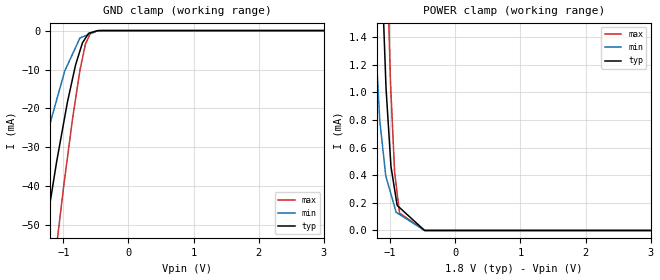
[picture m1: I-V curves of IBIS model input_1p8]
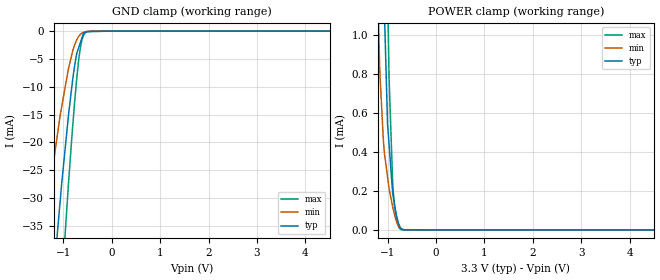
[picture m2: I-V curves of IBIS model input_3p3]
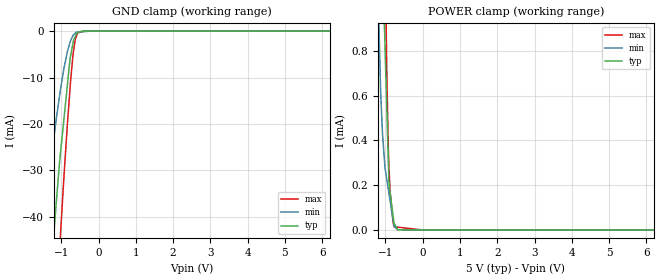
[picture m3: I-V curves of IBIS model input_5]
|Texas Instruments Incorporated
| Low-Power, 12-Bit, 1-MHz, Single/Dual Unipolar Input,
| ADCs with Serial Interface
| Marketing part#   Digital Voltage Range   Package-type   #pins
| ADS7229IPW   1.65V - 5.5V   TSSOP   16
| ADS7229IPWG4   1.65V - 5.5V   TSSOP   16
| ADS7229IPWR   1.65V - 5.5V   TSSOP   16
| ADS7229IPWRG4   1.65V - 5.5V   TSSOP   16
| ADS7229IRSAR   1.65V - 5.5V   QFN   16
| ADS7229IRSARG4   1.65V - 5.5V   QFN   16
| ADS7229IRSAT   1.65V - 5.5V   QFN   16
| ADS7229IRSATG4   1.65V - 5.5V   QFN   16
[IBIS Ver]   3.2
[File name]   ads7229.ibs
|SIMDE Ver   V3.0 - 201101 - RHL4 - Build 457
[File Rev]   1.0
[Date]   5/3/2011
[Source]
| Texas Instruments Incorporated.
| Analog-eLab Design Center, HPA
| 12500 TI Blvd
| Dallas, TX -75243
| e-mail: elab_ibis@list.ti.com
| -Model generated from simulations in TISPICE
[Notes]   Revision History:
| Rev 1.0: 5/3/2011
| - Initial version of the model
| - Model generated from simulations in TISPICE
| - Model matched to SPICE simulation
| - C_comp although listed in numerical order of value are
|   obtained from varying PVT conditions. For PVT conditions for
|   each specific value refer the buffer description under
|   respective [Model]. IBIS model user is responsible for using
|   appropriate C_comp to simulate for Signal Integrity.
| - Model names with a trailing _1p8 contains the model for
|   1.8V [1.71V and 1.89V].Model names with a trailing _3p3 contains
|   the model for 3.3V [3.0V and 3.6V].Model names with a trailing _5 contains
|   the model for 5.0V [4.5V and 5.5V].
[Disclaimer]
| This model is designed as an aid for customers of Texas Instruments.
| TI and its licensors and suppliers make no warranties, either expressed
| or implied, with respect to this  model, including the warranties of
| merchantability or fitness for a particular purpose. The model is
| provided solely on an "as is" basis. The entire risk as to its quality
| and performance is with the customer.
[Copyright]
 (C) Copyright 2011 Texas Instruments Incorporated.All rights reserved.
|   ADS7229PW
[Component]   ADS7229PW
[Manufacturer]   TI
[Package]   |16 TSSOP   -  PW package
|   typ   min   max
R_pkg   0.17749   0.15829   0.21843
L_pkg   2.44525nH   2.22777nH   3.33924nH
C_pkg   0.44775pF   0.43606pF   0.50175pF
[Pin]  signal_name   model_name   R_pin   L_pin   C_pin
1   +VA   POWER   0.07682   2.65655nH  0.56177pF
2   RESERVED   TERM   0.18443   2.44991nH  0.43771pF
3   +IN   TERM   0.16169   2.25622nH  0.44404pF
4   -IN   TERM   0.15829   2.22777nH  0.44306pF
5   AGND   GND   0.05843   1.75876nH  0.50047pF
6   REF-   TERM   0.16730   2.30339nH  0.44803pF
7   REF+(REFIN)   TERM   0.18343   2.44468nH  0.43606pF
8   NC   NC   0.01109   1.86891nH  0.43090pF
9   _CONVST   INPUT   0.21843   3.33924nH  0.50175pF
10   EOC/_INT/CDI   INT   0.19615   2.54951nH  0.44066pF
11   FS/_CS   INPUT   0.16617   2.29432nH  0.44526pF
12   SDI   INPUT   0.16006   2.24269nH  0.44303pF
13   SDO   SDO   0.16535   2.28523nH  0.44508pF
14   BDGND   GND   0.08779   1.96252nH  0.47461pF
15   SCLK   INPUT   0.19106   2.50478nH  0.44053pF
16   +VBD   POWER   0.11043   2.78979nH  0.53699pF
|   ADS7229RSA
[Component]   ADS7229RSA
[Manufacturer]   TI
[Package]   |16 QFN   -  RSA package
|   typ   min   max
R_pkg   0.06643   0.06002   0.07122
L_pkg   1.04867nH   0.94125nH   1.13043nH
C_pkg   0.15387pF   0.14348pF   0.16599pF
[Pin]  signal_name   model_name   R_pin   L_pin   C_pin
1   REF+(REFIN)   TERM   0.06354   1.00616nH  0.14531pF
2   NC   NC   0.00077   0.12730nH  0.10311pF
3   _CONVST   INPUT   0.06574   1.03694nH  0.16121pF
4   EOC/_INT/CDI   INT   0.06336   1.00311nH  0.14589pF
5   FS/_CS   INPUT   0.07094   1.12623nH  0.15264pF
6   SDI   INPUT   0.06830   1.07609nH  0.16380pF
7   SDO   SDO   0.07026   1.10762nH  0.16599pF
8   BDGND   GND   0.03616   0.81702nH  0.18339pF
9   SCLK   INPUT   0.06079   0.95368nH  0.14397pF
10   +VBD   POWER   0.03047   0.62846nH  0.18823pF
11   +VA   POWER   0.02067   0.54704nH  0.21082pF
12   RESERVED   TERM   0.06002   0.94125nH  0.14348pF
13   +IN   TERM   0.06902   1.09129nH  0.15099pF
14   -IN   TERM   0.06755   1.06261nH  0.16377pF
15   AGND   GND   0.02332   0.63786nH  0.22576pF
16   REF-   TERM   0.07122   1.13043nH  0.15551pF
|   Model Selectors
[Model Selector] INPUT
input_1p8  1.8V digital input
input_3p3  3.3V digital input
input_5   5.0V digital input
[Model Selector] INT
int_1p8  1.8V digital I/O
int_3p3  3.3V digital I/O
int_5   5.0V digital I/O
[Model Selector] SDO
sdo_1p8  1.8V digital 3-state output
sdo_3p3  3.3V digital 3-state output
sdo_5   5.0V digital 3-state output
[Model Selector] TERM
term_1-8V  1.8V nominal termination
term_3-3V  3.3V nominal termination
term_5-0V  5.0V nominal termination
[Model]  term_1-8V
Model_type Terminator
C_comp   1.0e-20F  1.0e-20F  1.0e-20F
|   typ   min   max
[Voltage Range]   1.8V   1.71V   1.89V
[POWER Clamp Reference]   1.8V   1.71V   1.89V
[GND Clamp Reference]   0V   0V   0V
|Ambient Temperature   25   85   -40
|Junction Temperature
[Temperature Range]   28   88   -40
[Model]  term_3-3V
Model_type Terminator
C_comp   1.0e-20F  1.0e-20F  1.0e-20F
|   typ   min   max
[Voltage Range]   3.3V   3.0V   3.6V
[POWER Clamp Reference]   3.3V   3.0V   3.6V
[GND Clamp Reference]   0V   0V   0V
|Ambient Temperature   25   85   -40
|Junction Temperature
[Temperature Range]   28   88   -40
[Model]  term_5-0V
Model_type Terminator
C_comp   1.0e-20F  1.0e-20F  1.0e-20F
|   typ   min   max
[Voltage Range]   5.0V   4.5V   5.5V
[POWER Clamp Reference]   5.0V   4.5V   5.5V
[GND Clamp Reference]   0V   0V   0V
|Ambient Temperature   25   85   -40
|Junction Temperature
[Temperature Range]   28   88   -40
| Models and submodels in the file (12): input_1p8 (Input), input_3p3 (Input), input_5 (Input), int_1p8 (I/O), int_3p3 (I/O), int_5 (I/O), sdo_1p8 (3-state), sdo_3p3 (3-state), sdo_5 (3-state), term_1-8V (Terminator), term_3-3V (Terminator), term_5-0V (Terminator)
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|   input_1p8 Model
[Model]   input_1p8
Model_type   Input
Vinl = 0.63
Vinh = 1.17
|   typ   min   max
|   (nom PVT)   (Fast PVT)   (slow PVT)
|C_comp from frequency sweep method(F=50MHz)
|Average
|C_comp   1.977e-12   1.603e-12   2.232e-12
|C_comp from L-C Tank method(L=1nH)
|Resonant Frequency(Hz)   3.960e9   4.380e9   3.660e9
C_comp   1.617e-12   1.322e-12   1.893e-12
| Where nom  PVT is Nominal Process,  1.8V,  28C
|   Fast PVT is Strong Process,   1.89V,  -40C
|   Slow PVT is Weak Process,   1.71V,  88C
[Model Spec]
|Subparameter   typ   min   max
Vinh   1.17   1.1115   1.2285
Vinl   0.63   0.5985   0.6615
[Voltage Range]   1.8   1.71   1.89
|Ambient Temperature   25   85   -40
|Junction Temperature
[Temperature Range]   28   88   -40
[Power Clamp Reference]   1.8   1.71   1.89
[GND Clamp Reference]   0   0   0
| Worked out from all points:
|   GND clamp passes 1 mA (typ) near -0.62 V on its own axis
|   POWER clamp passes 1 mA (typ) near -1.06 V on its own axis
[GND Clamp]
|   Voltage   I(typ)   I(min)   I(max)
-1.8V     -112.6mA   -67.57mA   -158.3mA
-1.71V    -101.8mA   -60.7mA    -144.9mA
-1.294V   -53.7mA    -29.29mA   -83.17mA
-1.103V   -33.79mA   -17.88mA   -55.3mA
-990.4mV  -23.34mA   -11.12mA   -39.49mA
-934.2mV  -18.18mA   -8.782mA   -32.36mA
-811.8mV  -8.843mA   -4.358mA   -17.59mA
-743.9mV  -5.179mA   -1.902mA   -10.17mA
-659.6mV  -1.956mA   -1.323mA   -3.452mA
-585.9mV  -566uA     -816.1uA   -753.5uA
-470.6mV  -24.01uA   -23.81uA   -26.74uA
3.6V      0A         0A         0A
[POWER Clamp]
|   Voltage   I(typ)   I(min)   I(max)
-1.8V     13.74mA    9.573mA    18.5mA
-1.249V   3.704mA    1.585mA    5.945mA
-1.158V   2.248mA    785.2uA    4.049mA
-1.1V     1.501mA    535.9uA    2.854mA
-1.062V   1.019mA    385.2uA    2.207mA
-997.9mV  537.6uA    279.6uA    1.113mA
-988.2mV  464.5uA    263.5uA    1.001mA
-931.8mV  297.1uA    170.5uA    422.6uA
-892.8mV  181.5uA    126.8uA    269.6uA
-856.2mV  165.7uA    115.8uA    125.7uA
-471.6mV  0A         407nA      322.8nA
3.6V      0A         0A         0A
|   input_3p3 Model
[Model]   input_3p3
Model_type   Input
Vinl = 1.155
Vinh = 2.145
|   typ   min   max
|   (nom PVT)   (Fast PVT)   (slow PVT)
|C_comp from frequency sweep method(F=50MHz)
|Average
|C_comp   1.787e-12   1.492e-12   2.072e-12
|C_comp from L-C Tank method(L=1nH)
|Resonant Frequency(Hz)   4.090e9   4.510e9   3.770e9
C_comp   1.516e-12   1.247e-12   1.784e-12
| Where nom  PVT is Nominal Process,  3.3V,  28C
|   Fast PVT is Strong Process,   3.6V,  -40C
|   Slow PVT is Weak Process,   3V,  88C
[Model Spec]
|Subparameter   typ   min   max
Vinh   2.145   1.95   2.34
Vinl   1.155   1.05   1.26
[Voltage Range]   3.3   3   3.6
|Ambient Temperature   25   85   -40
|Junction Temperature
[Temperature Range]   28   88   -40
[Power Clamp Reference]   3.3   3   3.6
[GND Clamp Reference]   0   0   0
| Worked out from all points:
|   GND clamp passes 1 mA (typ) near -0.61 V on its own axis
|   POWER clamp passes 1 mA (typ) near -1.05 V on its own axis
[GND Clamp]
|   Voltage   I(typ)   I(min)   I(max)
-3.3V     -299.5mA   -209.5mA   -377.4mA
-1.386V   -63.89mA   -35.54mA   -96.4mA
-1.198V   -43.41mA   -23.04mA   -68.75mA
-1.068V   -30.46mA   -15.1mA    -50.27mA
-1.033V   -27.06mA   -13.39mA   -45.32mA
-897.6mV  -15.17mA   -6.745mA   -27.5mA
-778.8mV  -6.771mA   -2.72mA    -13.72mA
-726mV    -4.006mA   -1.559mA   -8.502mA
-684mV    -2.903mA   -926.5uA   -5.026mA
-591mV    -462.9uA   -220.2uA   -913.4uA
-378mV    -81uA      -1.882uA   -1.021uA
6.6V      0A         0A         0A
[POWER Clamp]
|   Voltage   I(typ)   I(min)   I(max)
-3.3V     43.07mA    34.83mA    54.13mA
-1.211V   3.046mA    1.261mA    5.284mA
-1.164V   2.375mA    827uA      4.3mA
-1.089V   1.315mA    458.5uA    2.733mA
-1.055V   1.008mA    371uA      2.019mA
-1.003V   546.1uA    273.1uA    1.247mA
-896.4mV  188.2uA    118.2uA    239.9uA
-860.4mV  129.5uA    82.19uA    134.9uA
-813.6mV  69.71uA    40.8uA     54.22uA
-766.8mV  29.28uA    16.98uA    12.79uA
-709.2mV  4.986uA    4.596uA    1.015uA
6.6V      0A         0A         0A
|   input_5 Model
[Model]   input_5
Model_type   Input
Vinl = 1.75
Vinh = 3.25
|   typ   min   max
|   (nom PVT)   (Fast PVT)   (slow PVT)
|C_comp from frequency sweep method(F=50MHz)
|Average
|C_comp   1.734e-12   1.407e-12   1.985e-12
|C_comp from L-C Tank method(L=1nH)
|Resonant Frequency(Hz)   4.190e9   4.610e9   3.860e9
C_comp   1.444e-12   1.193e-12   1.702e-12
| Where nom  PVT is Nominal Process,  5V,  28C
|   Fast PVT is Strong Process,   5.5V,  -40C
|   Slow PVT is Weak Process,   4.5V,  88C
[Model Spec]
|Subparameter   typ   min   max
Vinh   3.25   2.925   3.575
Vinl   1.75   1.575   1.925
[Voltage Range]   5   4.5   5.5
|Ambient Temperature   25   85   -40
|Junction Temperature
[Temperature Range]   28   88   -40
[Power Clamp Reference]   5   4.5   5.5
[GND Clamp Reference]   0   0   0
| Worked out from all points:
|   GND clamp passes 1 mA (typ) near -0.62 V on its own axis
|   POWER clamp passes 1 mA (typ) near -1.04 V on its own axis
[GND Clamp]
|   Voltage   I(typ)   I(min)   I(max)
-5V       -511.9mA   -383.6mA   -620.3mA
-1.602V   -89.09mA   -51.94mA   -128.6mA
-1.375V   -62.65mA   -34.77mA   -94.77mA
-1.188V   -42.46mA   -22.2mA    -67.28mA
-1.026V   -26.63mA   -12.83mA   -44.4mA
-841.5mV  -12.03mA   -4.604mA   -20.73mA
-753.5mV  -5.488mA   -2.139mA   -11.11mA
-682mV    -2.441mA   -906.6uA   -4.884mA
-598.5mV  -719.6uA   -250.5uA   -1.219mA
-561mV    -290.8uA   -226.8uA   -397.3uA
-390.5mV  -7.937uA   -118.9uA   -1.624uA
10V       0A         0A         0A
[POWER Clamp]
|   Voltage   I(typ)   I(min)   I(max)
-5V       76.86mA    64.15mA    94.96mA
-1.183V   2.644mA    969.1uA    4.554mA
-1.08V    1.211mA    430.1uA    2.483mA
-1.012V   822.9uA    277.5uA    1.325mA
-1.001V   756.8uA    265.1uA    1.157mA
-962.5mV  535.2uA    223.7uA    683.9uA
-924mV    313.6uA    182.4uA    372.9uA
-905mV    204.3uA    161.9uA    277.3uA
-874.5mV  164.9uA    129.2uA    169.7uA
-770mV    29.83uA    16.87uA    14.44uA
-670.5mV  1.356uA    960.3nA    12.58uA
10V       0A         0A         0A
